VAR_GLOBAL
	AxisArray					: ARRAY [1..7] OF Axis_REF;
	IsMaterialDown              : BOOL;
	MaterialNum                 : INT;
	BeltAxis                    : Axis_ref;//皮带轴
	REALBeltAxis                : Axis_ref;//皮带轴
	 // 机器人变量
	(*in_stKinToPlc	AT %I*		: NcToPlc_NciChannel_Ref;
	out_stPlcToKin	AT %Q*		: PLCTONC_NCICHANNEL_REF;*)
	stKinToPlc	AT %I*		    : NcToPlc_NciChannel_Ref;
	stPlcToKin	AT %Q*		    : PLCTONC_NCICHANNEL_REF;
END_VAR
